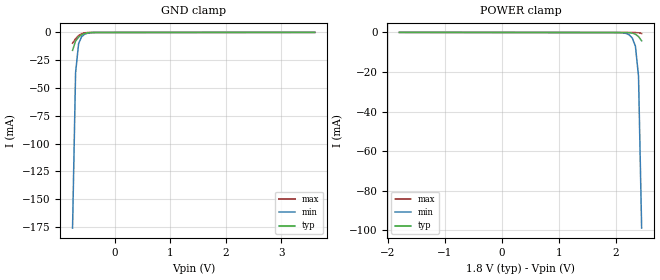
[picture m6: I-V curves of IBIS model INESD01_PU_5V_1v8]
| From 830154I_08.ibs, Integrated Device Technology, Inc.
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[Model] INESD01_PU_5V_1v8
Model_type   Input
Polarity   Non-Inverting
Vinl = 0.63V
Vinh = 1.17V
|   typ   min   max
C_comp   2pF   1.5pF   2.5pF
|   typ   min   max
[Voltage range]   1.8V   1.710V   1.89V
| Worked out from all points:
|   GND clamp passes 1 mA (typ) near -0.55 V on its own axis
[GND_clamp]
|Voltage   I (typ)   I (min)   I (max)
|Note, modeling breaks down at 250mA and above.  This is well beyond the functional   |
|operating range of the device.  Should this scenario occur, catastrophic failure and   |
|possible damage to the device and/or board is of higher concern than the I-V curve   |
|behavior.  The IBIS checker will flag currents in excess of 10A with warnings.  Lines   |
|with currents in excess of 0.35 A have been commented out.  The points still remain|
|available to the user if the user desires to use them.   |
|-1.80000e+00   -1.13308e+01   -1.03205e+01   -1.30899e+01
|-1.74545e+00   -1.06865e+01   -9.78359e+00   -1.22674e+01
|-1.69091e+00   -1.00423e+01   -9.24667e+00   -1.14448e+01
|-1.63636e+00   -9.39807e+00   -8.70978e+00   -1.06223e+01
|-1.58182e+00   -8.75387e+00   -8.17292e+00   -9.79976e+00
|-1.52727e+00   -8.10970e+00   -7.63610e+00   -8.97723e+00
|-1.47273e+00   -7.46555e+00   -7.09932e+00   -8.15471e+00
|-1.41818e+00   -6.82145e+00   -6.56260e+00   -7.33220e+00
|-1.36364e+00   -6.17740e+00   -6.02593e+00   -6.50972e+00
|-1.30909e+00   -5.53340e+00   -5.48933e+00   -5.68727e+00
|-1.25455e+00   -4.88948e+00   -4.95282e+00   -4.86488e+00
|-1.20000e+00   -4.24564e+00   -4.41640e+00   -4.04254e+00
|-1.14545e+00   -3.60190e+00   -3.88009e+00   -3.22028e+00
|-1.09091e+00   -2.95829e+00   -3.34390e+00   -2.39813e+00
|-1.03636e+00   -2.31484e+00   -2.80787e+00   -1.57612e+00
|-9.81818e-01   -1.67156e+00   -2.27200e+00   -7.54281e-01
|-9.27273e-01   -1.02854e+00   -1.73636e+00   -1.06718e-01
|-8.72727e-01   -3.85796e-01   -1.20097e+00   -2.52183e-02
|-8.18182e-01   -5.97690e-02   -6.65862e-01   -1.48435e-02
-763.6mV  -16.14mA   -176.1mA   -9.719mA
-709.1mV  -7.75mA    -36.23mA   -5.703mA
-654.5mV  -4.239mA   -10.04mA   -2.781mA
-600mV    -2.093mA   -3.835mA   -1.079mA
-545.5mV  -878.8uA   -1.65mA    -351.1uA
-490.9mV  -326.8uA   -685.6uA   -115.4uA
-327.3mV  -45.76uA   -69.92uA   -33.79uA
3.6V      35.07uA    46.05uA    25.82uA
[Power_clamp]
|Voltage   I (typ)   I (min)   I (max)
|Note, modeling breaks down at 250mA and above.  This is well beyond the functional   |
|operating range of the device.  Should this scenario occur, catastrophic failure and   |
|possible damage to the device and/or board is of higher concern than the I-V curve   |
|behavior.  The IBIS checker will flag currents in excess of 10A with warnings.  Lines   |
|with currents in excess of 0.35 A have been commented out.  The points still remain|
|available to the user if the user desires to use them.   |
-1.8V     35.07uA    43.86uA    27.17uA
2.018V    -39.45uA   -61.93uA   -30.47uA
2.127V    -45.76uA   -203uA     -32.12uA
2.236V    -125.4uA   -1.222mA   -34.43uA
2.291V    -326.8uA   -2.848mA   -39.62uA
2.345V    -878.8uA   -6.968mA   -64.62uA
2.4V      -2.093mA   -22.19mA   -167.4uA
2.455V    -4.239mA   -98.94mA   -525.8uA
